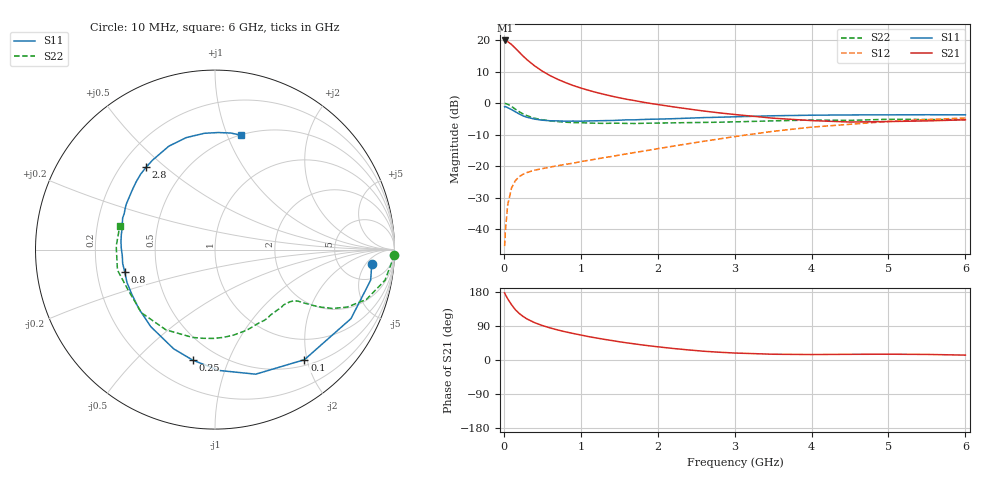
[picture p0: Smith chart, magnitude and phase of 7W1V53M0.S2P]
! Infineon Technologies  Discrete & RF Semiconductors
! BFS17W
! Si NPN RF Bipolar Junction Transistor in SOT323
! VCE = 1.5 V  IC = 3 mA
! Common Emitter S-Parameters:  August  1999
# GHz  S  MA  R  50
!  f  S11  S21  S12  S22
! GHz  MAG  ANG  MAG  ANG  MAG  ANG  MAG  ANG
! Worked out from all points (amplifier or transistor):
!   36 points, 10 MHz to 6 GHz, reference 50 ohm
!   highest |S21| = 19.9 dB at 20 MHz (marker M1)
!   |S21| within 3 dB of that: start of sweep to 171.4 MHz
!   unconditionally stable (mu >= 1): 664.7 MHz to end of sweep
!   at 250 MHz: K = 0.46, MSG = 18.7 dB, |S12| = -22.5 dB
!   at 1.4 GHz: K = 1.34, MAG = 6.1 dB, |S12| = -16.9 dB
!   at 6 GHz: K = 1.11, MAG = -2.3 dB, |S12| = -4.7 dB
!   S11 on the Smith chart (normalised r, x): 10 MHz: 10, -7; 100 MHz: 0.60, -1.95; 250 MHz: 0.37, -0.75; 800 MHz: 0.32, -0.11; 2.8 GHz: 0.30, +0.43; 6 GHz: 0.51, +1.12
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0.01  0.8769 -5.3  9.81 177.0  0.0054 85.6  0.9951 -1.6
0.02  0.8839 -11.1  9.87 172.6  0.0095 86.1  0.9868 -4.2
0.05  0.8496 -26.9  9.464 161.6  0.0244 75.6  0.9626 -10.2
0.1  0.7903 -50.9  8.525 145.9  0.0452 64.2  0.8884 -18.2
0.15  0.7302 -71.9  7.423 132.7  0.0591 54.9  0.803 -23.5
0.2  0.6737 -88.1  6.444 122.8  0.0684 49.5  0.7324 -26.6
0.25  0.6281 -101.4  5.583 114.9  0.0746 45.0  0.6743 -28.4
0.3  0.599 -112.6  4.9 108.5  0.0795 43.1  0.6348 -29.5
0.4  0.5588 -129.9  3.904 98.5  0.0866 40.5  0.5764 -31.0
0.5  0.5372 -142.2  3.221 91.0  0.0916 40.4  0.545 -31.8
0.6  0.526 -151.8  2.739 84.7  0.0969 41.3  0.5234 -33.0
0.8  0.5181 -166.0  2.122 74.4  0.1071 43.3  0.4993 -36.8
0.9  0.5201 -171.5  1.908 70.0  0.1116 45.2  0.4912 -38.8
1.1  0.5224 179.0  1.6 61.8  0.1239 47.6  0.4845 -43.8
1.3  0.5285 171.0  1.383 54.7  0.1367 50.0  0.4781 -49.6
1.6  0.544 161.0  1.151 45.2  0.1573 53.1  0.4768 -58.4
2.2  0.5671 144.7  0.875 30.4  0.208 57.0  0.4875 -77.8
2.8  0.5984 129.8  0.702 20.5  0.2708 57.0  0.4989 -98.0
3.5  0.6312 114.0  0.578 15.2  0.3577 52.7  0.524 -121.4
4.5  0.6507 95.3  0.502 15.0  0.4627 41.2  0.5338 -155.0
5.5  0.6555 82.2  0.523 14.7  0.548 29.6  0.5506 177.9
6  0.6532 77.1  0.545 12.9  0.5825 24.0  0.5466 165.9
